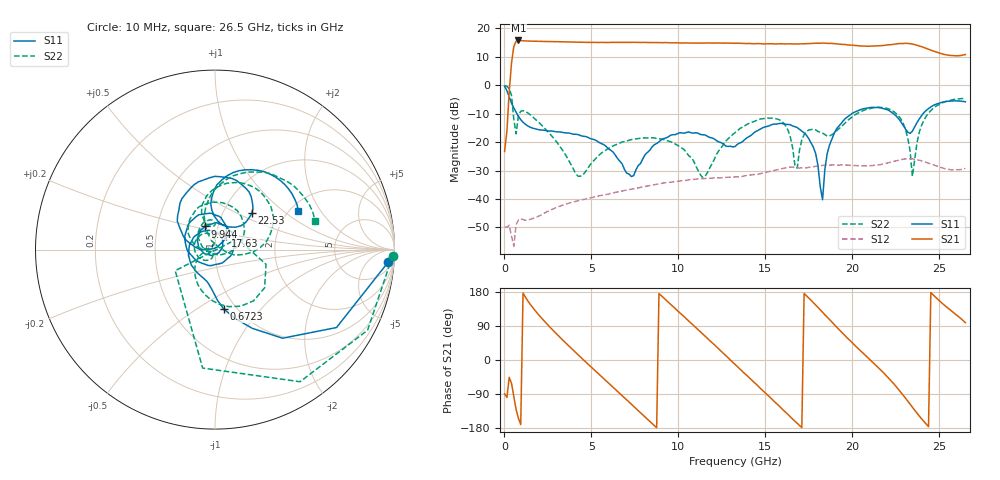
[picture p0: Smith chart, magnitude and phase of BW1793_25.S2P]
!Agilent Technologies,N5242A,MY52422126,A.09.90.01
!Agilent N5242A: A.09.90.01
!Date: Wednesday, September 07, 2016 19:45:58
!Correction: S11(Full 2 Port(1,2))
!S21(Full 2 Port(1,2))
!S12(Full 2 Port(1,2))
!S22(Full 2 Port(1,2))
!S2P File: Measurements: S11, S21, S12, S22:
# Hz S  dB  R 50
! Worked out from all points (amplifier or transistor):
!   201 points, 10 MHz to 26.5 GHz, reference 50 ohm
!   highest |S21| = 15.8 dB at 804.7 MHz (marker M1)
!   |S21| within 3 dB of that: 519.2 MHz to 24.35 GHz (23.83 GHz wide, 192 % of centre)
!   unconditionally stable (mu >= 1): start of sweep to end of sweep
!   at 4.381 GHz: K = 9.08, MAG = 15.2 dB, |S12| = -40.5 dB
!   at 13.26 GHz: K = 3.72, MAG = 14.9 dB, |S12| = -32.3 dB
!   at 26.5 GHz: K = 2.41, MAG = 13.4 dB, |S12| = -29.3 dB
!   S11 on the Smith chart (normalised r, x): 10 MHz: 10, -23; 672.2 MHz: 0.88, -0.65; 9.944 GHz: 0.87, +0.23; 17.63 GHz: 1.12, +0.17; 22.53 GHz: 1.36, +0.60; 26.5 GHz: 2.20, +1.29
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1e7  -0.29 -4.2  -23.26 -89.3  -49.91 -1.3  -0.09 -2.0
4.0735e8  -6.28 -64.7  7.84 -61.6  -53.10 -35.5  -3.56 -96.0
6.7225e8  -9.50 -81.5  15.51 -131.1  -49.01 32.7  -17.10 25.8
8.047e8  -10.92 -87.0  15.77 -154.2  -47.35 15.5  -10.58 -16.1
1.46695e9  -14.71 -103.9  15.54 148.0  -47.20 -5.6  -10.30 -85.5
2.3941e9  -15.95 -134.0  15.42 97.6  -44.65 -19.2  -15.63 -133.0
4.5133e9  -17.93 133.6  15.12 1.5  -40.22 -80.7  -31.52 -121.0
6.76495e9  -27.64 12.8  15.10 -93.8  -37.22 -151.2  -19.97 -153.9
8.88415e9  -19.93 159.9  15.02 175.4  -34.65 134.6  -18.82 135.7
9.94375e9  -17.05 113.3  14.94 130.2  -33.76 94.6  -21.07 105.8
1.14007e10  -17.41 49.2  14.85 68.8  -32.86 38.5  -32.48 123.7
1.3255e10  -21.57 -89.6  14.79 -11.4  -32.29 -32.3  -16.67 156.8
1.524175e10  -14.20 142.6  14.63 -97.2  -30.29 -106.4  -11.57 87.7
1.64338e10  -13.88 95.1  14.59 -149.8  -28.76 -160.1  -18.19 6.6
1.762585e10  -20.25 51.4  14.73 157.7  -28.79 150.8  -15.58 105.6
1.77583e10  -21.77 46.5  14.78 151.3  -28.65 145.7  -15.46 99.0
1.948015e10  -12.46 146.9  14.38 69.2  -27.96 69.8  -13.91 110.8
2.080465e10  -8.10 98.9  13.75 9.9  -28.37 17.3  -8.49 79.6
2.212915e10  -8.96 55.5  14.25 -50.1  -27.15 -34.0  -8.41 32.1
2.25265e10  -10.83 44.6  14.59 -70.4  -26.54 -53.1  -9.99 14.9
2.398345e10  -10.67 93.5  13.59 -155.3  -26.60 -137.4  -14.06 107.7
2.65e10  -5.83 25.1  10.81 98.6  -29.27 118.9  -4.72 15.8
